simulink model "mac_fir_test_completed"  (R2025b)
settings: Solver=VariableStepDiscrete  StartTime=0.0  StopTime=2500  RelTol=1e-3
undefined symbols (not defined in the file or in its folder): A, B, code, Convert_config, Evaluation, ffva1156, gateway_in_config, gateway_out_config, hex2dec, KCU105, Kintex, P, Platform, sysgen, UltraScale, xcku040
libraries: hdlBasic x7, simulink x2, vmcUtilities x1, hdlDSPIP x1

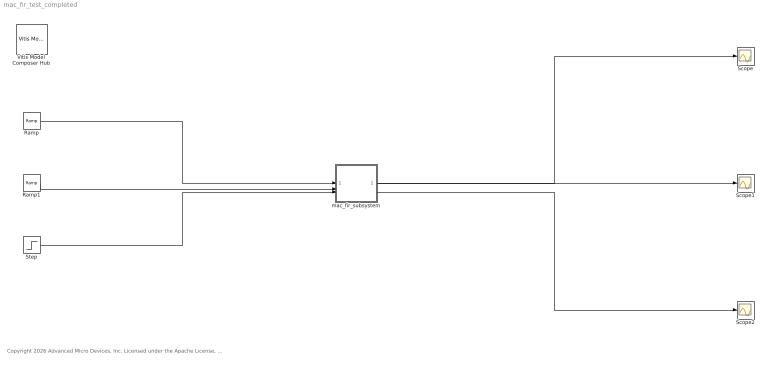
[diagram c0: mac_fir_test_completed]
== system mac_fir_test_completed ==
  note: Copyright 2026 Advanced Micro Devices, Inc. Licensed under the Apache License, Version 2.0 (the "License"); you may not use this file except in compliance with the License. You may obtain a copy of the License at http://www.apache.org/licenses/LICENSE-2.0 Unless required by applicable law or agreed to in writing, software distributed under the License is distributed on an "AS IS" BASIS, WITHOUT WARRANTIES OR CONDITIONS OF ANY KIND, either express or implied. See the License for the specific language governing permissions and limitations under the License.
  Ramp : simulink/Sources/Ramp  slope=1  start=0  InitialOutput=0
  Ramp1 : simulink/Sources/Ramp  slope=1  start=0  InitialOutput=0
  Scope : Scope
  Scope1 : Scope
  Scope2 : Scope
  Step : Step  Before=1  After=0  SampleTime=0
  Vitis Model Composer Hub : vmcUtilities/Vitis Model Composer Hub  Tag=genX  CodeGeneration=off  StartColumn=1  NumberOfColumns=1  TargetDirectory=./code  exportDesign=off  analyzeDesign=off  validateDesignOnHw=off  ExportType=AI Engines  IpVendor=xilinx.com  IpLibrary=hls  IpVersion=1.0  IpHWLanguage=Verilog  AieCompilerOptions={}  AieSimulatorOptions={}  CreateTestbench=off  TestbenchStackSize=10  RunRtlSim=off  RunCSim=off  RunAieSim=off  AieSimTimeout=50000  RunAieSimProfiling=off  LaunchVitisAnalyzer=off  PlotOutput=off  RunX86Sim=off  X86SimTimeout=10  GenHwImage=off  GenLibadfXo=off  GenHwValidationCode=off  PlatformType=Not Specified  HwSystemType=Baremetal  HwValidationTarget=hw  ProjDevice=Kintex-UltraScale KCU105 Evaluation Platform (xcku040-ffva1156-2-e)  ProjDevicePart=xcku040-ffva1156-2-e  AIEType=None  SamplePeriod=-1  ClockFrequency=200  DataPathParallelism=1  xilinxfamily=kintexu  part=xcku040  speed=-2-e  package=ffva1156  directory=./code  testbench=off  incr_netlist=off  synthesis_tool=Vivado  clock_wrapper=Clock Enables  dbl_ovrd=According to Block Masks  dcm_input_clock_period=10  sysclk_period=10  simulink_period=1  eval_field=0  LogFileName=''  NThreads=4
  mac_fir_subsystem : Subsystem
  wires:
  Ramp/1 -> mac_fir_subsystem/1(In1)
  Ramp1/1 -> mac_fir_subsystem/2(In2)
  Step/1 -> mac_fir_subsystem/3(In3)
  mac_fir_subsystem/1(Out1) -> Scope/1
  mac_fir_subsystem/2(Out2) -> Scope1/1
  mac_fir_subsystem/3(Out3) -> Scope2/1

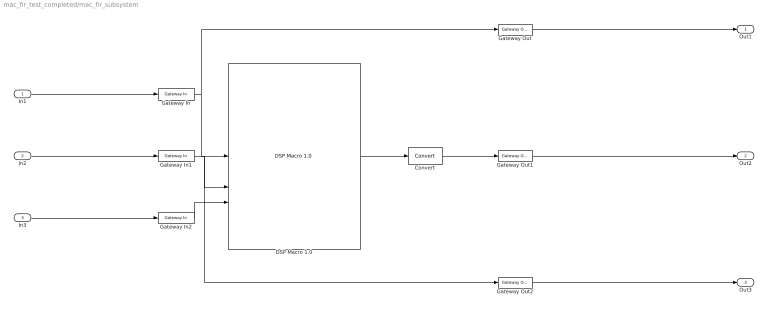
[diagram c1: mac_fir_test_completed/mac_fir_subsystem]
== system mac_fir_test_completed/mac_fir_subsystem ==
  In1 : Inport
  In2 : Inport  Port=2
  In3 : Inport  Port=3
  Convert : hdlBasic/Convert  gui_display_data_type=Fixed-point  arith_type="Signed  (2's comp)"  n_bits=27  bin_pt=0  float_type=Single  exp_bits=8  fraction_bits=24  quantization=Truncate  overflow=Wrap  en=off  latency=0  pipeline=off  XmcBlockStatus=1  maskContainerNames=group2  block_type=convert  block_config=sysgen:Convert_config  block_width=595  block_height=885
  DSP Macro 1.0 : hdlDSPIP/DSP Macro 1.0   dsptype=Target XtremeDSP Slice: DSP48E1  instruction_list=A*B+P  AvailableInstructions=|  show_filtered=off  pipeline_options=Automatic  tier_1=off  tier_2=off  tier_3=off  tier_4=off  tier_5=off  tier_6=off  dreg_1=off  dreg_2=off  dreg_3=off  areg_1=off  areg_2=off  areg_3=on  areg_4=on  breg_1=off  breg_2=off  breg_3=on  breg_4=on  mreg_5=on  concatreg_3=off  concatreg_4=off  concatreg_5=off  creg_1=off  creg_2=off  creg_3=off  creg_4=off  creg_5=off  preg_6=on  cinreg_1=off  cinreg_2=off  cinreg_3=off  cinreg_4=off  cinreg_5=off  opreg_1=off  opreg_2=off  opreg_3=on  opreg_4=on  opreg_5=on  output_properties=Full_Precision  p_width=48  p_binarywidth=0  has_acout=off  has_bcout=off  has_pcout=off  has_carryout=off  has_carrycascout=off  has_ce=off  has_d_ce=off  has_a_ce=off  has_b_ce=off  has_concat_ce=off  has_c_ce=off  has_m_ce=off  has_p_ce=off  has_sel_ce=off  has_sclr=on  has_d_sclr=off  has_a_sclr=off  has_b_sclr=off  has_concat_sclr=off  has_c_sclr=off  has_m_sclr=off  has_p_sclr=off  has_sel_sclr=off  use_dsp48=on  XmcBlockStatus=1  maskContainerNames=Container4  simulation_type=xsim  gui_behaviour=Sysgen  instruction1='#'  ip_name=DSP Macro  ip_version=1.0  dsptool_ready=true  ipcore_usecache=true  ipcore_useipmodelcache=true  wrapper_available=true  port_translation_map={ 'ce' => 'en', 'sclr' => 'rst'}  ipcore_latency_function='has_combinational'  structural_sim=false  ipcore_verbose=false  ipcore_port_config={ 'carryin' => { 'arith' => 'ufix', 'binpt' => 0.00000000000, 'width' => 1.00000000000}, 'carrycascin' => { 'arith' => 'ufix', 'binpt' => 0.00000000000, 'width' => 1.00000000000}, 'carrycascout' => { 'arith' => 'ufix', 'binpt' => 0.00000000000, 'width' => 1.00000000000}, 'carryout' => { 'arith' => 'ufix', 'binpt' => 0.00000000000, 'width' => 1.00000000000}}  ipcore_xco_need_fpga_part=true  ipcore_fpga_part=[]  block_type=dsp_macro_v1_0
      | #
      | (A+D)
      | (A+D)*B
      | (A+D)*B+C
      | (A+D)*B+C+CARRYIN
      | (A+D)*B+CARRYIN
      | (A+D)*B+P
      | (A+D)*B+P+CARRYIN
      | (A+D)*B+P>>17
      | (A+D)*B+P>>17+CARRYIN
      | (A+D)*B+PCIN
      | (A+D)*B+PCIN+CARRYIN
      | (A+D)*B+PCIN>>17
      | (A+D)*B+PCIN>>17+CARRYIN
      | (A+D)*B-C
      | (A+D)*B-P
      | (A+D)*B-P>>17
      | (A+D)*B-PCIN
      | (A+D)*B-PCIN>>17
      | (A+D)*BCIN
      | (A+D)*BCIN+C
      | (A+D)*BCIN+C+CARRYIN
      | (A+D)*BCIN+CARRYIN
      | (A+D)*BCIN+P
      | (A+D)*BCIN+P+CARRYIN
      | (A+D)*BCIN+P>>17
      | (A+D)*BCIN+P>>17+CARR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
  Gateway In : hdlBasic/Gateway In  gui_display_data_type=Fixed-point  arith_type=Signed (2's comp)  n_bits=8  bin_pt=0  preci_type=Single  exp_width=8  frac_width=24  rows=1  columns=1  quantization="Round  (unbiased: +/- Inf)"  overflow=Saturate  period=1  UseAsADC=off  ADCChannel='1'  interface=None  automatic_assignment=on  address_offset=hex2dec('00')  intf_name=''  intf_description=''  default_value=0  timing_constraint=None  locs_specified=off  LOCs={}  io_standard={}  inherit_from_input=off  hdl_port=on  XmcBlockStatus=1  maskContainerNames=group4  block_type=gatewayin  block_config=sysgen:gateway_in_config  block_width_w=590  block_height_w=620  block_width=640  block_height=850
  Gateway In1 : hdlBasic/Gateway In  gui_display_data_type=Fixed-point  arith_type=Signed (2's comp)  n_bits=12  bin_pt=0  preci_type=Single  exp_width=8  frac_width=24  rows=1  columns=1  quantization="Round  (unbiased: +/- Inf)"  overflow=Saturate  period=1  UseAsADC=off  ADCChannel='1'  interface=None  automatic_assignment=on  address_offset=hex2dec('00')  intf_name=''  intf_description=''  default_value=0  timing_constraint=None  locs_specified=off  LOCs={}  io_standard={}  inherit_from_input=off  hdl_port=on  XmcBlockStatus=1  maskContainerNames=group4  block_type=gatewayin  block_config=sysgen:gateway_in_config  block_width_w=590  block_height_w=620  block_width=640  block_height=850
  Gateway In2 : hdlBasic/Gateway In  gui_display_data_type=Boolean  arith_type=Boolean  n_bits=16  bin_pt=14  preci_type=Single  exp_width=8  frac_width=24  rows=1  columns=1  quantization="Round  (unbiased: +/- Inf)"  overflow=Saturate  period=1  UseAsADC=off  ADCChannel='1'  interface=None  automatic_assignment=on  address_offset=hex2dec('00')  intf_name=''  intf_description=''  default_value=0  timing_constraint=None  locs_specified=off  LOCs={}  io_standard={}  inherit_from_input=off  hdl_port=on  XmcBlockStatus=1  maskContainerNames=group4  block_type=gatewayin  block_config=sysgen:gateway_in_config  block_width_w=590  block_height_w=620  block_width=640  block_height=850
  Gateway Out : hdlBasic/Gateway Out  inherit_from_input=off  bool_to_boolean=off  hdl_port=off  rows=1  columns=1  UseAsDAC=off  DACChannel='1'  interface=None  automatic_assignment=on  address_offset=hex2dec('00')  intf_name=''  intf_description=''  timing_constraint=None  locs_specified=off  LOCs={}  io_standard={}  XmcBlockStatus=1  maskContainerNames=group4  block_type=gatewayout  block_config=sysgen:gateway_out_config  block_width_w=590  block_height_w=620  block_width=620  block_height=750
  Gateway Out1 : hdlBasic/Gateway Out  inherit_from_input=off  bool_to_boolean=off  hdl_port=on  rows=1  columns=1  UseAsDAC=off  DACChannel='1'  interface=None  automatic_assignment=on  address_offset=hex2dec('00')  intf_name=''  intf_description=''  timing_constraint=None  locs_specified=off  LOCs={}  io_standard={}  XmcBlockStatus=1  maskContainerNames=group4  block_type=gatewayout  block_config=sysgen:gateway_out_config  block_width_w=590  block_height_w=620  block_width=620  block_height=750
  Gateway Out2 : hdlBasic/Gateway Out  inherit_from_input=off  bool_to_boolean=off  hdl_port=off  rows=1  columns=1  UseAsDAC=off  DACChannel='1'  interface=None  automatic_assignment=on  address_offset=hex2dec('00')  intf_name=''  intf_description=''  timing_constraint=None  locs_specified=off  LOCs={}  io_standard={}  XmcBlockStatus=1  maskContainerNames=group4  block_type=gatewayout  block_config=sysgen:gateway_out_config  block_width_w=590  block_height_w=620  block_width=620  block_height=750
  Out1 : Outport
  Out2 : Outport  Port=2
  Out3 : Outport  Port=3
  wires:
  Gateway Out2/1 -> Out3/1
  DSP Macro 1.0/1 -> Convert/1
  Gateway In2/1 -> DSP Macro 1.0/3
  In3/1 -> Gateway In2/1
  In2/1 -> Gateway In1/1
  Convert/1 -> Gateway Out1/1
  Gateway In/1 -> Gateway Out/1, DSP Macro 1.0/1
  Gateway Out1/1 -> Out2/1
  Gateway Out/1 -> Out1/1
  Gateway In1/1 -> Gateway Out2/1, DSP Macro 1.0/2
  In1/1 -> Gateway In/1
